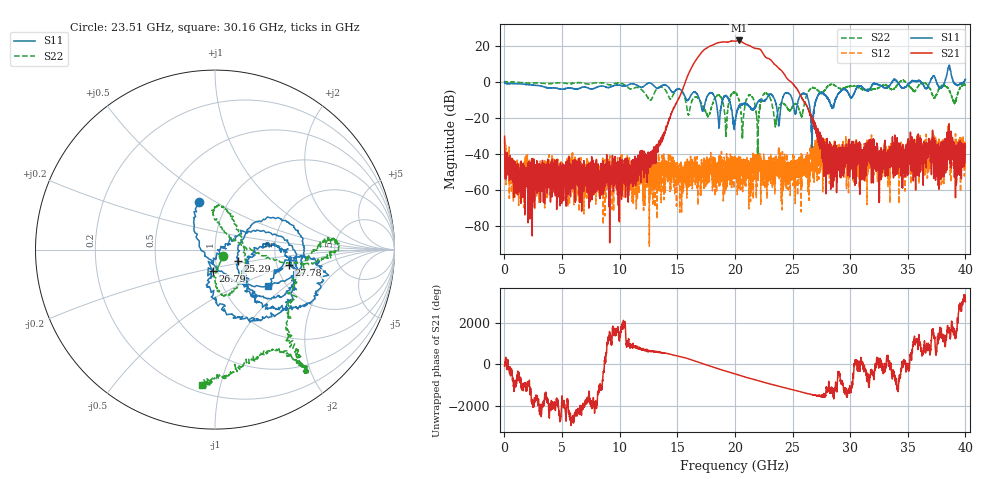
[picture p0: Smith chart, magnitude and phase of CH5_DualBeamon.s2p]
!Keysight Technologies,N5245B,MY57181321,A.14.80.03
!Date: Thursday, March 28, 2024 18:53:17
!Correction: S11(C  2-Port  )
!S21(C  2-Port  )
!S12(C  2-Port  )
!S22(C  2-Port  )
!S2P File: Measurements: S11, S21, S12, S22:
# Hz S  RI  R 50
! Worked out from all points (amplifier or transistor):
!   4000 points, 10 MHz to 40 GHz, reference 50 ohm
!   highest |S21| = 22.8 dB at 20.33 GHz (marker M1)
!   |S21| within 3 dB of that: 17.87 GHz to 21.3 GHz (3.427 GHz wide, 17.5 % of centre)
!   unconditionally stable (mu >= 1): 19.77 MHz to 33.65 GHz; 36.12 GHz to 36.94 GHz; 38.97 GHz to 39.89 GHz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
!   at 6.67 GHz: K = 2710.15, MAG = -38.5 dB, |S12| = -48.2 dB
!   at 20.01 GHz: K = 8.50, MAG = 23.7 dB, |S12| = -49.6 dB
!   at 40 GHz: K = -230.33, MSG = 0.0 dB, |S12| = -35.8 dB
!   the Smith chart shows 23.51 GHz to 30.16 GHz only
!   S11 on the Smith chart (normalised r, x): 23.51 GHz: 0.74, +0.42; 25.29 GHz: 1.28, -0.16; 26.79 GHz: 0.95, -0.22; 27.78 GHz: 2.33, -0.49; 30.16 GHz: 1.62, -0.76
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1e7  1.006 -0.0467  0.0013 -0.0309  0.0258 0.00553  -0.9411 0.0129
6.68e9  0.5071 0.4707  0.000712 0.00188  -0.00322 0.00193  0.9278 0.0879
1.334e10  -0.5977 -0.2743  -0.0128 -0.00698  -0.00106 0.00488  -0.6795 -0.0683
1.703e10  0.2019 0.148  1.993 5.687  -0.00215 -1.5e-05  0.1307 0.2319
1.749e10  0.2302 -0.2078  7.878 -2.503  -0.000359 -0.0073  -0.1085 0.0824
1.794e10  0.4686 -0.1705  -1.581 -9.839  -0.00319 0.00213  0.0303 -0.1791
1.844e10  0.1955 0.0352  -11.55 1.814  -9.2e-05 0.00431  0.3867 -0.1501
1.893e10  -0.0751 -0.3137  1.249 12.49  0.00128 -0.00308  0.277 0.0169
1.949e10  0.2019 -0.2454  12.54 -1.603  -0.00255 -0.00173  -0.2121 -0.1818
2.001e10  -0.0409 0.0606  -1.3 -13.17  -0.00332 3.81e-05  -0.2351 -0.4431
2.033e10  -0.1838 -0.12  -12.09 -6.707  -0.00564 0.00634  -0.0777 -0.3031
2.092e10  0.2051 -0.1452  -3.328 10.43  0.000861 -0.00286  -0.1031 0.2416
2.152e10  -0.0621 0.1567  8.572 2.671  -0.00248 0.00308  -0.3028 0.2173
2.214e10  -0.1286 -0.2869  0.9953 -7.988  0.00573 -0.0021  0.199 0.00129
2.351e10  -0.0866 0.264  0.8489 2.758  0.0018 0.00494  0.046 -0.0359
2.529e10  0.1256 -0.0622  -0.685 -0.0155  0.00311 0.0049  0.0138 0.2399
2.667e10  0.0284 -0.00123  0.0875 -0.0213  0.00112 -0.00327  0.6521 -0.0118
2.679e10  -0.0132 -0.117  0.0805 -0.0413  -0.00197 0.000324  0.669 0.0375
2.778e10  0.4125 -0.0869  -0.00275 -0.0216  -0.0119 -0.00484  0.4044 -0.396
3.016e10  0.2957 -0.2032  -0.00487 0.00153  -0.00246 -0.00504  -0.0729 -0.7554
3.334e10  0.1735 -0.7013  0.00258 0.0033  -0.00953 -0.0106  -0.3486 -0.6127
4e10  -0.8782 -0.7568  -0.0136 0.00879  -0.00188 -0.0161  0.4902 0.6368
